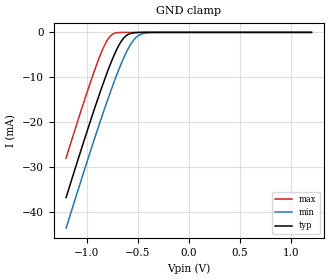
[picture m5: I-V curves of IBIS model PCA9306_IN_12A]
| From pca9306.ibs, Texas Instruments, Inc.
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[Model]   PCA9306_IN_12A
Model_type  Input
Vinl=0.6
Vinh=1.2
| variable   typ   min   max
C_comp   5.55pF   4.55pF   7.53pF
[Temperature Range]   40   100   -40
| Ambient temperature   25   85   -40
[Voltage range]   1.2   1.2   1.2
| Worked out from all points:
|   GND clamp passes 1 mA (typ) near -0.62 V on its own axis
[GND Clamp]
| PCA9306_IN_12A
|   Voltage   I(typ)   I(min)   I(max)
-1.2V     -36.82mA   -43.65mA   -28.01mA
-945mV    -18.59mA   -25.32mA   -9.995mA
-865mV    -13.2mA    -19.8mA    -5.032mA
-805mV    -9.368mA   -15.79mA   -2.046mA
-745mV    -5.864mA   -11.94mA   -415.1uA
-695mV    -3.367mA   -8.913mA   -66.15uA
-650mV    -1.659mA   -6.397mA   -10.67uA
-575mV    -291.5uA   -2.917mA   -462.9nA
-505mV    -38.56uA   -933.2uA   -24.98nA
-445mV    -6.068uA   -254.4uA   -2.07nA
-345mV    -270.4nA   -21.14uA   -35.62pA
1.2V      25.7pA     2.801nA    17.46pA
